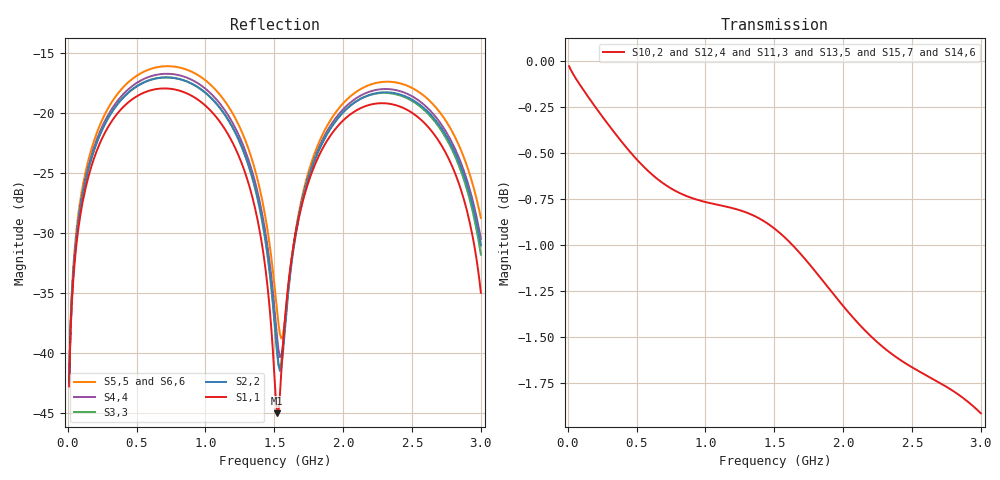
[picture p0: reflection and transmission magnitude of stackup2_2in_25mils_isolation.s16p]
! Touchstone file from project
# GHZ S RI R 50.000000
! Modal data exported
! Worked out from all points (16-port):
!   300 points, 10 MHz to 3 GHz, reference 50 ohm
!   strongest paths, dB at 10 MHz, 760 MHz, 1.51 GHz, 2.26 GHz, 3 GHz:
!     S10,2: 0.0, -0.7, -0.9, -1.5, -1.9
!     S12,4: 0.0, -0.7, -0.9, -1.6, -1.9
!     S11,3: 0.0, -0.7, -0.9, -1.5, -1.9
!     S13,5: 0.0, -0.7, -0.9, -1.6, -1.9
!     S15,7: 0.0, -0.7, -0.9, -1.5, -1.9
!     S14,6: 0.0, -0.7, -0.9, -1.6, -1.9
!   lowest |S11| = -45.1 dB at 1.52 GHz (marker M1), VSWR 1.01, Z = 50.5 - j0.166 ohm
!   |S11| at or under -10 dB: start of sweep to end of sweep
